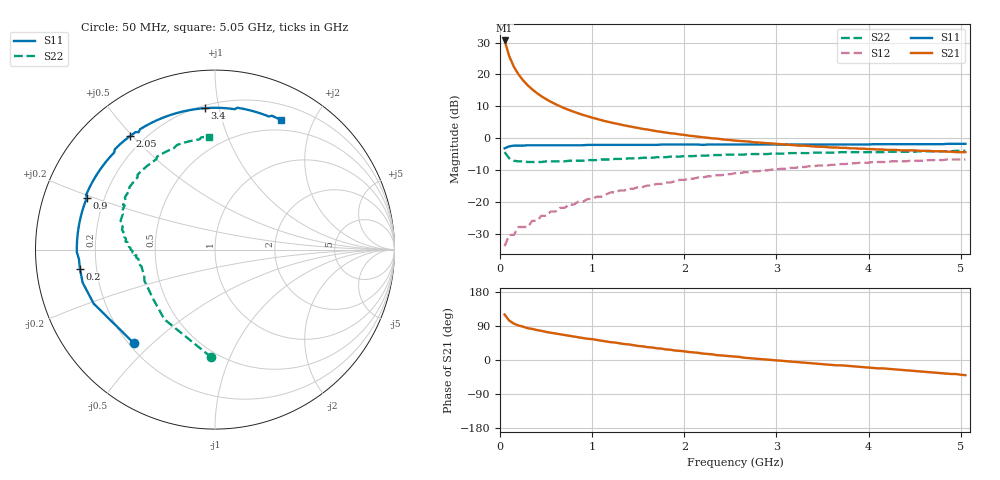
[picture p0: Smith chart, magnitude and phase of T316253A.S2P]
!AT-31625
!S-PARAMETERS at Vce=3.0 V  Ic=50 mA.  LAST UPDATED 08-05-96
# ghz s ma r 50
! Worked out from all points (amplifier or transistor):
!   101 points, 50 MHz to 5.05 GHz, reference 50 ohm
!   highest |S21| = 30.7 dB at 50 MHz (marker M1)
!   |S21| within 3 dB of that: start of sweep to 80.31 MHz
!   unconditionally stable (mu >= 1): 494.2 MHz to 512.8 MHz; 568.6 MHz to 1.198 GHz; 1.203 GHz to 1.48 GHz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
!   at 850 MHz: K = 1.03, MAG = 12.7 dB, |S12| = -20.0 dB
!   at 2.55 GHz: K = 0.93, MSG = 5.1 dB, |S12| = -11.1 dB
!   at 5.05 GHz: K = 0.96, MSG = 1.2 dB, |S12| = -6.7 dB
!   S11 on the Smith chart (normalised r, x): 50 MHz: 0.22, -0.44; 200 MHz: 0.14, -0.07; 900 MHz: 0.13, +0.19; 2.05 GHz: 0.15, +0.49; 3.4 GHz: 0.22, +0.91; 5.05 GHz: 0.37, +1.57
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0.05  0.69 -131.0  34.12 120.0  0.02 42.0  0.6 -92.0
0.1  0.74 -156.0  19.3 104.0  0.03 37.0  0.48 -126.0
0.15  0.76 -166.0  13.22 96.0  0.03 40.0  0.44 -142.0
0.2  0.76 -172.0  10.03 91.0  0.04 44.0  0.43 -151.0
0.25  0.76 -176.0  8.08 88.0  0.04 47.0  0.43 -156.0
0.3  0.77 -179.0  6.75 84.0  0.04 50.0  0.42 -160.0
0.35  0.77 178.0  5.81 82.0  0.05 53.0  0.42 -163.0
0.4  0.77 176.0  5.09 79.0  0.05 55.0  0.42 -165.0
0.45  0.77 173.0  4.53 77.0  0.06 56.0  0.42 -167.0
0.5  0.77 171.0  4.09 74.0  0.06 57.0  0.43 -169.0
0.55  0.77 170.0  3.72 72.0  0.07 58.0  0.43 -170.0
0.65  0.77 166.0  3.16 68.0  0.08 59.0  0.43 -172.0
0.75  0.77 163.0  2.75 64.0  0.09 60.0  0.44 -174.0
0.9  0.77 158.0  2.31 58.0  0.1 60.0  0.44 -176.0
1.2  0.78 150.0  1.76 47.0  0.14 58.0  0.46 -179.0
1.5  0.78 141.0  1.44 37.0  0.17 54.0  0.48 177.0
1.75  0.79 135.0  1.25 30.0  0.19 51.0  0.5 174.0
2.05  0.79 127.0  1.09 21.0  0.23 46.0  0.52 169.0
2.55  0.79 114.0  0.91 9.0  0.28 38.0  0.55 161.0
3.4  0.79 94.0  0.74 -9.0  0.36 22.0  0.59 144.0
4.25  0.8 78.0  0.65 -24.0  0.43 3.0  0.61 120.0
5.05  0.81 63.0  0.6 -40.0  0.46 -14.0  0.63 93.0
